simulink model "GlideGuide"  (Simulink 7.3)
settings: Solver=ode45  StartTime=0.0  StopTime=10.0  RelTol=1e-3
undefined symbols (not defined in the file or in its folder): kh, khd, khi

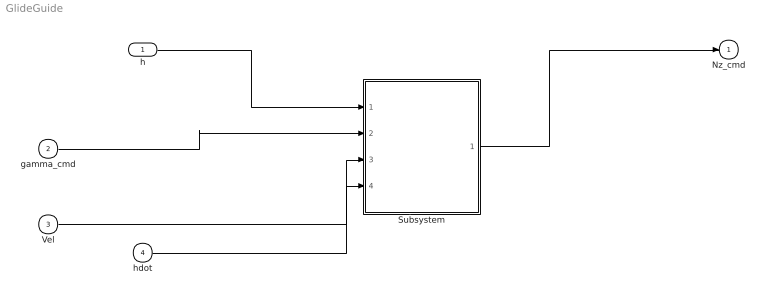
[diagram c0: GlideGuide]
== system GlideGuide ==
  h : Inport  OutDataType=sfix(16)  OutScaling=2^0
  gamma_cmd : Inport  Port=2  OutDataType=sfix(16)  OutScaling=2^0
  Vel : Inport  Port=3  OutDataType=sfix(16)  OutScaling=2^0
  hdot : Inport  Port=4  OutDataType=sfix(16)  OutScaling=2^0
  Subsystem : Subsystem
  Nz_cmd : Outport  InitialOutput=0
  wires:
  h/1 -> Subsystem/1(h)
  Subsystem/1(Nz_cmd) -> Nz_cmd/1
  gamma_cmd/1 -> Subsystem/2(gamma_cmd)
  Vel/1 -> Subsystem/3(Vel)
  hdot/1 -> Subsystem/4(hdot)

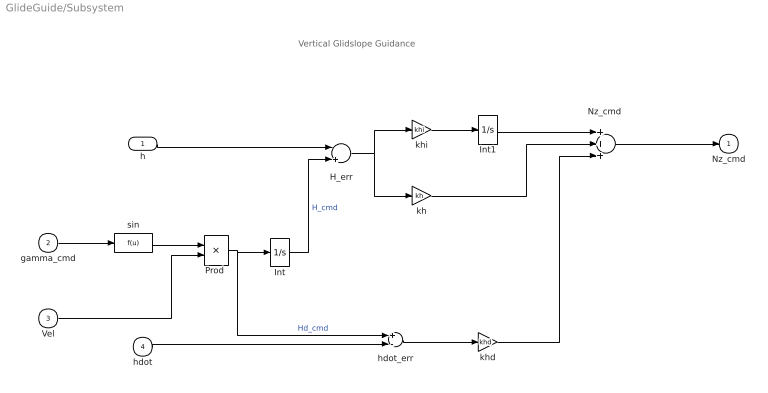
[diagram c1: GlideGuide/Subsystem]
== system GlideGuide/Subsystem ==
  note: Vertical Glidslope Guidance
  h : Inport  OutDataType=sfix(16)  OutScaling=2^0
  gamma_cmd : Inport  Port=2  OutDataType=sfix(16)  OutScaling=2^0
  Vel : Inport  Port=3  OutDataType=sfix(16)  OutScaling=2^0
  hdot : Inport  Port=4  OutDataType=sfix(16)  OutScaling=2^0
  H_err : Sum  Inputs=-+  OutDataType=sfix(16)  OutScaling=2^0
  Int : Integrator
  Int1 : Integrator
  "Nz_cmd " : Sum  Inputs=+++  OutDataType=sfix(16)  OutScaling=2^0
  "Prod " : Product  OutDataType=sfix(16)  OutScaling=2^0
  hdot_err : Sum  Inputs=+-  OutDataType=sfix(16)  OutScaling=2^0
  kh : Gain  Gain=kh  ParameterDataType=sfix(16)  ParameterScaling=2^0  OutDataType=sfix(16)  OutScaling=2^0
  khd : Gain  Gain=khd  ParameterDataType=sfix(16)  ParameterScaling=2^0  OutDataType=sfix(16)  OutScaling=2^0
  khi : Gain  Gain=khi  ParameterDataType=sfix(16)  ParameterScaling=2^0  OutDataType=sfix(16)  OutScaling=2^0
  sin : Fcn
  Nz_cmd : Outport  InitialOutput=0
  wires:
  "Nz_cmd "/1 -> Nz_cmd/1
  h/1 -> H_err/1
  gamma_cmd/1 -> sin/1
  sin/1 -> "Prod "/1
  "Prod "/1 -> Int/1, hdot_err/1  "Hd_cmd"
  Vel/1 -> "Prod "/2
  khi/1 -> Int1/1
  H_err/1 -> khi/1, kh/1
  Int1/1 -> "Nz_cmd "/1
  kh/1 -> "Nz_cmd "/2
  khd/1 -> "Nz_cmd "/3
  hdot/1 -> hdot_err/2
  hdot_err/1 -> khd/1
  Int/1 -> H_err/2  "H_cmd"
